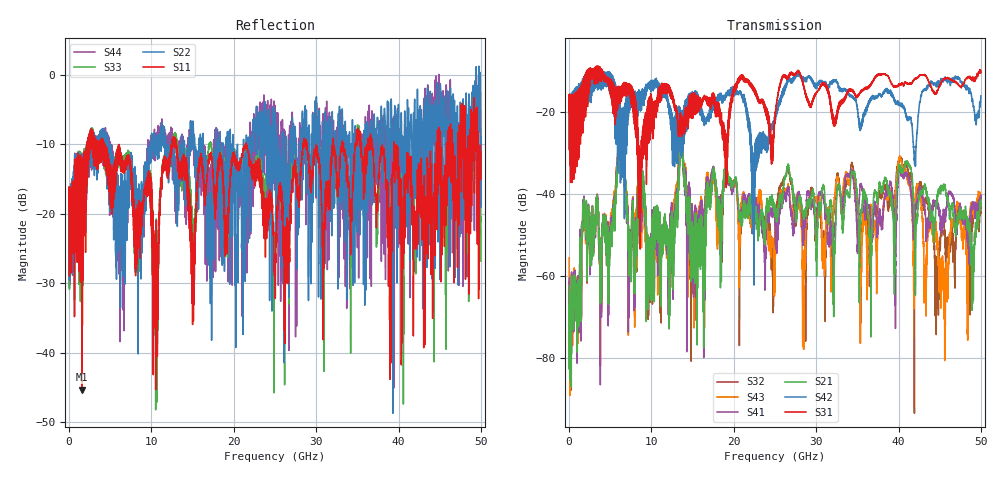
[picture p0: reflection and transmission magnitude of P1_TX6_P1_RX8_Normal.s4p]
!Keysight Technologies,N5225B,MY57041031,A.13.20.10
!Date: Friday, May 31, 2019 11:26:09
!Correction: S11(Full 4 Port(1,2,3,4))
!S12(Full 4 Port(1,2,3,4))
!S13(Full 4 Port(1,2,3,4))
!S14(Full 4 Port(1,2,3,4))
!S21(Full 4 Port(1,2,3,4))
!S22(Full 4 Port(1,2,3,4))
!S23(Full 4 Port(1,2,3,4))
!S24(Full 4 Port(1,2,3,4))
!S31(Full 4 Port(1,2,3,4))
!S32(Full 4 Port(1,2,3,4))
!S33(Full 4 Port(1,2,3,4))
!S34(Full 4 Port(1,2,3,4))
!S41(Full 4 Port(1,2,3,4))
!S42(Full 4 Port(1,2,3,4))
!S43(Full 4 Port(1,2,3,4))
!S44(Full 4 Port(1,2,3,4))
!S4P File: Measurements: <S11,S12,S13,S14>,
!<S21,S22,S23,S24>,
!<S31,S32,S33,S34>,
!<S41,S42,S43,S44>:
# Hz S  dB  R 50.0
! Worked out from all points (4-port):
!   5000 points, 10 MHz to 50 GHz, reference 50 ohm
!   strongest paths, dB at 10 MHz, 12.51 GHz, 25.01 GHz, 37.51 GHz, 50 GHz:
!     S31: -19.4, -15.5, -21.6, -10.8, -9.9
!     S42: -19.4, -24.4, -22.4, -16.1, -16.0
!     S21: -62.5, -44.4, -44.1, -41.1, -41.3
!     S41: -60.5, -43.4, -44.8, -47.8, -40.2
!     S43: -55.5, -44.8, -55.1, -46.0, -40.8
!     S32: -61.3, -45.6, -47.7, -42.5, -43.4
!   lowest |S11| = -45.3 dB at 1.57 GHz (marker M1), VSWR 1.01, Z = 49.5 - j0.0332 ohm
!   |S11| at or under -10 dB: 4.286 GHz to 12.47 GHz (8.179 GHz wide, 97.6 % of centre); 13.02 GHz to 21.43 GHz (8.402 GHz wide, 48.8 % of centre); 21.46 GHz to 28.42 GHz (6.959 GHz wide, 27.9 % of centre)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
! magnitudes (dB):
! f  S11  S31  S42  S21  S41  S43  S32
! 10 MHz  -19.4  -19.4  -19.4  -62.5  -60.5  -55.5  -61.3
! 1.57 GHz  -45.3  -22.2  -15.9  -47.5  -47.5  -47.0  -47.3
! 13.58 GHz  -14.3  -21.2  -22.1  -27.9  -26.9  -26.8  -27.6
! 28.49 GHz  -10.3  -13.9  -12.2  -46.1  -49.1  -62.1  -46.4
! 40.21 GHz  -21.6  -13.4  -18.1  -33.1  -34.2  -31.3  -31.4
! 45.73 GHz  -21.7  -11.8  -11.7  -39.8  -44.4  -61.4  -56.9
! 50 GHz  -11.1  -9.9  -16.0  -41.3  -40.2  -40.8  -43.4
